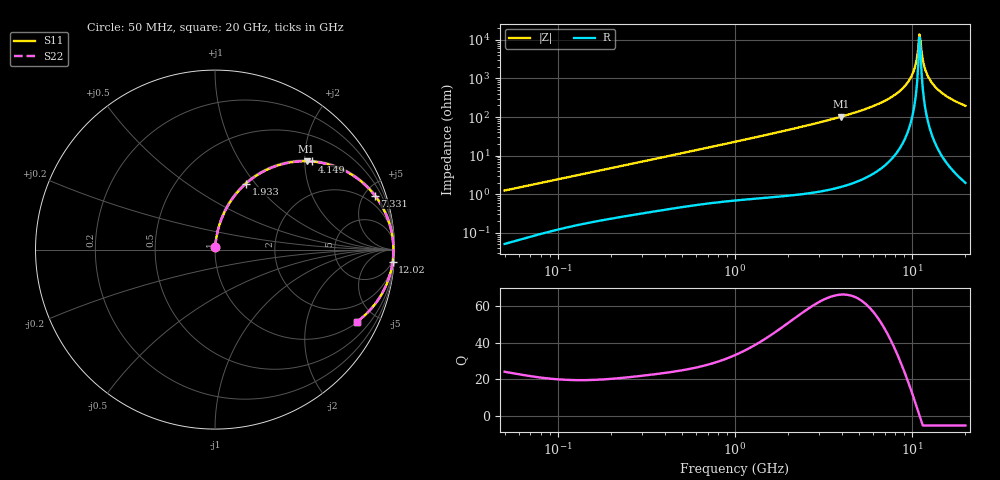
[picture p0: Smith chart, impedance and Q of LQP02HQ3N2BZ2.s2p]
!Murata Part Number: LQP02HQ3N2BZ2
!These Parameters are Measured in Series Mode Connection
!  o--[Z]--o
!Port1  Port2
!  o-------o
!Freq. Start=50[MHz] Stop=20[GHz], 401[Steps]
# Hz S RI R 50
!Freq.(Hz) S11(Real) S11(Imag) S21(Real) S21(Imag) S12(Real) S12(Imag) S22(Real) S22(Imag)
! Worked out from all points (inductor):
!   401 points, 50 MHz to 20 GHz, reference 50 ohm
!   read as one part in series: L = 3.95 nH near 51.52 MHz
!   highest Q = 66.1 at 3.967 GHz (marker M1), where L = 4.1 nH
!   self-resonance near 10.99 GHz
!   S11 on the Smith chart (normalised r, x): 50 MHz: 1.00, +0.02; 1.933 GHz: 1.02, +0.90; 4.149 GHz: 1.03, +2.17; 7.331 GHz: 1.13, +5.88; 12.02 GHz: 3, -29; 20 GHz: 1.04, -3.93
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5e7  0.000672 0.0125  0.9993 -0.0125  0.9993 -0.0125  0.000672 0.0125
1.364002e8  0.00275 0.0327  0.9973 -0.0327  0.9973 -0.0327  0.00275 0.0327
3.721004e8  0.0111 0.0854  0.9889 -0.0854  0.9889 -0.0854  0.0111 0.0854
1e9  0.0556 0.2145  0.9444 -0.2145  0.9444 -0.2145  0.0556 0.2145
1.932977e9  0.1724 0.3678  0.8276 -0.3678  0.8276 -0.3678  0.1724 0.3678
2.728004e9  0.3015 0.4506  0.6985 -0.4506  0.6985 -0.4506  0.3015 0.4506
3.967106e9  0.5105 0.4924  0.4895 -0.4924  0.4895 -0.4924  0.5105 0.4924
4.149438e9  0.5394 0.4909  0.4606 -0.4909  0.4606 -0.4909  0.5394 0.4909
5.683258e9  0.7466 0.4266  0.2534 -0.4266  0.2534 -0.4266  0.7466 0.4266
7.331367e9  0.8908 0.3007  0.1092 -0.3007  0.1092 -0.3007  0.8908 0.3007
7.442007e9  0.8978 0.2915  0.1022 -0.2915  0.1022 -0.2915  0.8978 0.2915
8.774992e9  0.96 0.1785  0.04 -0.1785  0.04 -0.1785  0.96 0.1785
9.745021e9  0.9837 0.0988  0.0163 -0.0988  0.0163 -0.0988  0.9837 0.0988
1.034674e10  0.9911 0.0516  0.00889 -0.0516  0.00889 -0.0516  0.9911 0.0516
1.082228e10  0.9937 0.0158  0.00633 -0.0158  0.00633 -0.0158  0.9937 0.0158
1.098561e10  0.9939 0.00389  0.00605 -0.00389  0.00605 -0.00389  0.9939 0.00389
1.131968e10  0.9936 -0.02  0.00636 0.02  0.00636 0.02  0.9936 -0.02
1.166392e10  0.9922 -0.0439  0.00783 0.0439  0.00783 0.0439  0.9922 -0.0439
1.201863e10  0.9895 -0.0677  0.0105 0.0677  0.0105 0.0677  0.9895 -0.0677
1.295331e10  0.978 -0.1263  0.022 0.1263  0.022 0.1263  0.978 -0.1263
1.438523e10  0.9504 -0.2047  0.0496 0.2047  0.0496 0.2047  0.9504 -0.2047
2e10  0.7916 -0.4012  0.2084 0.4012  0.2084 0.4012  0.7916 -0.4012
